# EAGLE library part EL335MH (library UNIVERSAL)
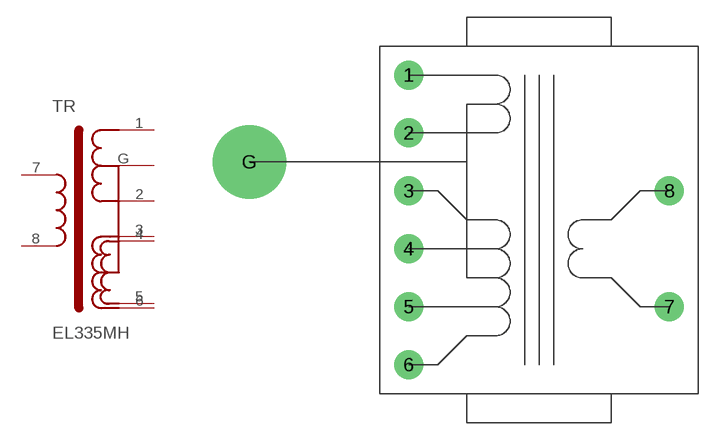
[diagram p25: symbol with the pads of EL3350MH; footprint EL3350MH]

Designator prefix TR

## EL335MH  [EL3350MH]
1  1
2  2
3  3
4  4
5  5
6  6
7  7
8  8
G  G

## Footprint EL3350MH (pad centres in mm)
drill 0.8 pad 2.54: 1 0,25.4; 2 0,20.32; 3 0,15.24; 4 0,10.16; 5 0,5.08; 6 0,0; 7 22.86,5.08; 8 22.86,15.24
drill 3.2 pad 6.452: G -13.97,17.78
